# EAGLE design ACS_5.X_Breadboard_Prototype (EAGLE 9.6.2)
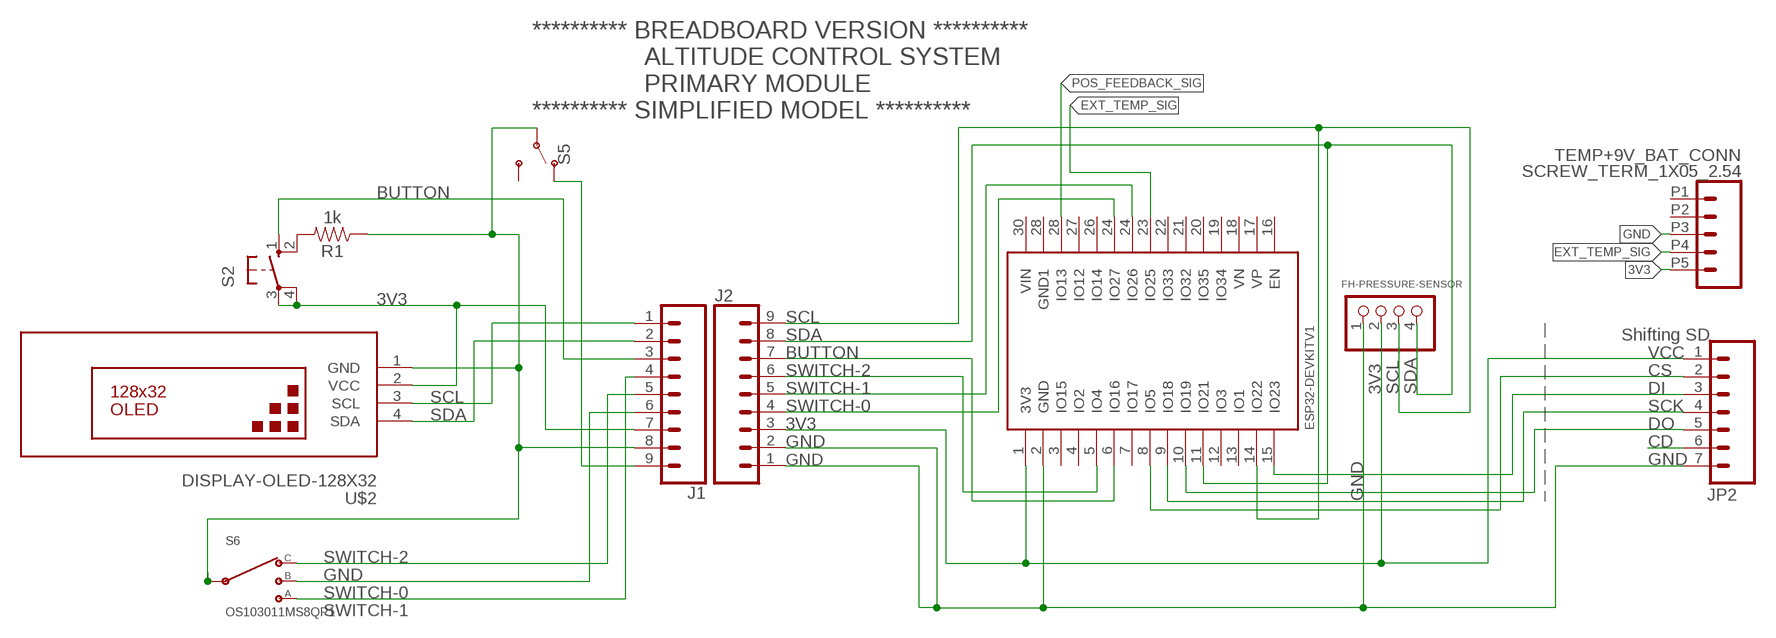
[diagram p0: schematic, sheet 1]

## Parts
FH-PRESSURE-SENSOR  PINHD-1X4  [1X04]
J1  CONN_09  [1X09]
J2  CONN_09  [1X09]
JP2  M07  [1X07]
R1  1k  1KOHM-HORIZ-1/4W-1%  [AXIAL-0.3]
S2  10-XX  [B3F-10XX]
S5  SWITCH-SPDT-PTH-11.6X4.0MM  [SWITCH_SPDT_PTH_11.6X4.0MM]
S6  OS103011MS8QP1  [OS102011MS8QP1]
TEMP+9V_BAT_CONN  SCREW_TERM_1X05_2.54  [1X05_2.54_SCREWTERM]
U$2  DISPLAY-OLED-128X32  [DISPLAY-OLED-128X32]
U$3  ESP32DEVKITV1  [ESP32-DEVKITV1]

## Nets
3V3: FH-PRESSURE-SENSOR.2 J1.7 J2.3 JP2.1 S2.3(P) S2.4(P1) TEMP+9V_BAT_CONN.P5 U$2.2(VCC) U$3.1(3V3)
BUTTON: J1.3 J2.7 S2.1(S) U$3.6(IO16)
EXT_TEMP_SIG: TEMP+9V_BAT_CONN.P4 U$3.23(IO25)
GND: FH-PRESSURE-SENSOR.1 J1.8 J2.1 J2.2 JP2.7 R1.P$1 S5.2(P) S6.2(C) TEMP+9V_BAT_CONN.P3 U$2.1(GND) U$3.2(GND)
N$1: R1.P$2 S2.2(S1)
N$4: J1.9 S5.1(O)
N$8: JP2.6
N$11: JP2.3 U$3.15(IO23)
N$12: JP2.2 U$3.8(IO5)
N$13: JP2.4 U$3.9(IO18)
N$14: JP2.5 U$3.10(IO19)
POS_FEEDBACK_SIG: U$3.28(IO13)
SCL: FH-PRESSURE-SENSOR.3 J1.1 J2.9 U$2.3(SCL) U$3.14(IO22)
SDA: FH-PRESSURE-SENSOR.4 J1.2 J2.8 U$2.4(SDA) U$3.11(IO21)
SWITCH-0: J1.6 J2.4 S6.3 U$3.24(IO27)
SWITCH-1: J1.5 J2.5 S6.4 U$3.24(IO26)
SWITCH-2: J1.4 J2.6 S6.1 U$3.5(IO4)
Unconnected: S5.3(S) TEMP+9V_BAT_CONN.P1 TEMP+9V_BAT_CONN.P2 U$3.3(IO15) U$3.4(IO2) U$3.7(IO17) U$3.12(IO3) U$3.13(IO1) U$3.16(EN) U$3.17(VP) U$3.18(VN) U$3.19(IO34) U$3.20(IO35) U$3.21(IO32) U$3.22(IO33) U$3.26(IO14) U$3.27(IO12) U$3.28(GND1) U$3.30(VIN)

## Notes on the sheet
- ********** BREADBOARD VERSION ********** 
                  ALTITUDE CONTROL SYSTEM
                  PRIMARY MODULE
  ********** SIMPLIFIED MODEL **********
- Shifting SD
- VCC
- CS
- DI
- SCK
- DO
- CD

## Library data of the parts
FH-PRESSURE-SENSOR = pinhead:PINHD-1X4: PIN HEADER
J1 J2 = SparkFun-Connectors:CONN_09: Multi connection point. Often used as Generic Header-pin footprint for 0.1 inch spaced/style header connections On any of the 0.1 inch spaced packages, you can populate with these: Break Away Headers - Straight (PRT-00116) Break Away Male Headers - Right Angle (PRT-00553) Female Headers (PRT-00115)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
JP2 = SparkFun-Connectors:M07: Header 7 Standard 7-pin 0.1" header. Use with straight break away headers (SKU : PRT-00116), right angle break away headers (PRT-00553), swiss pins (PRT-00743), machine pins (PRT-00117), and female headers (PRT-00115). NOTES ON THE VARIANTS LOCK and LOCK_LONGPADS... This footprint was designed to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
R1 = SparkFun-Resistors:1KOHM: 1kΩ resistor; PROD_ID: RES-12182
S2 = DC_LOAD_AU:10-XX: OMRON SWITCH; MPN: B3F-1000; OC_FARNELL: 176432; OC_NEWARK: 36M3542
S5 = SparkFun-Switches:SWITCH-SPDT: Single Pole, Double Throw (SPDT) Switch Single-pole, double-throw (SPDT) switch. Variant Overview SMD-AYZ0202 Surface Mount DPDT Switch (COM-00597) Used on e.g. LilyPad Arduino USB - ATmega32U4 Board PTH-11.6X4.0MM SPDT Mini Power Switch (COM-00102) Used on e.g. SparkFun Simon Says - Through-Hole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; PROD_ID: SWCH-08261; SF_SKU: COM-00102
S6 = OS103011MS8QP1:OS103011MS8QP1: Slide Switch SP3T Through Hole; AVAILABILITY: Unavailable; DESCRIPTION: Switch Slide ON ON ON SP3T Top Slide 0.1A 12VDC 10000Cycle PC Pins Bracket Mount/Through Hole Bulk; MF: C&K; MP: OS103011MS8QP1; PACKAGE: None; PRICE: None
TEMP+9V_BAT_CONN = Connectors-Terminal_Block:SCREW_TERM_1X05_2.54
U$2 = diy-modules:DISPLAY-OLED-128X32: 128x32 Dot Matrix OLED Module with I2C interface based on SSD1306 chip More details available here: http://www.tinyosshop.com/index.php?route=product/product&product_id=953 Schematic available here: http://www.tinyosshop.com/datasheet/OLED%2012832.pdf SSD1306 datasheet: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
U$3 = ESP32-DEVKITV1:ESP32DEVKITV1

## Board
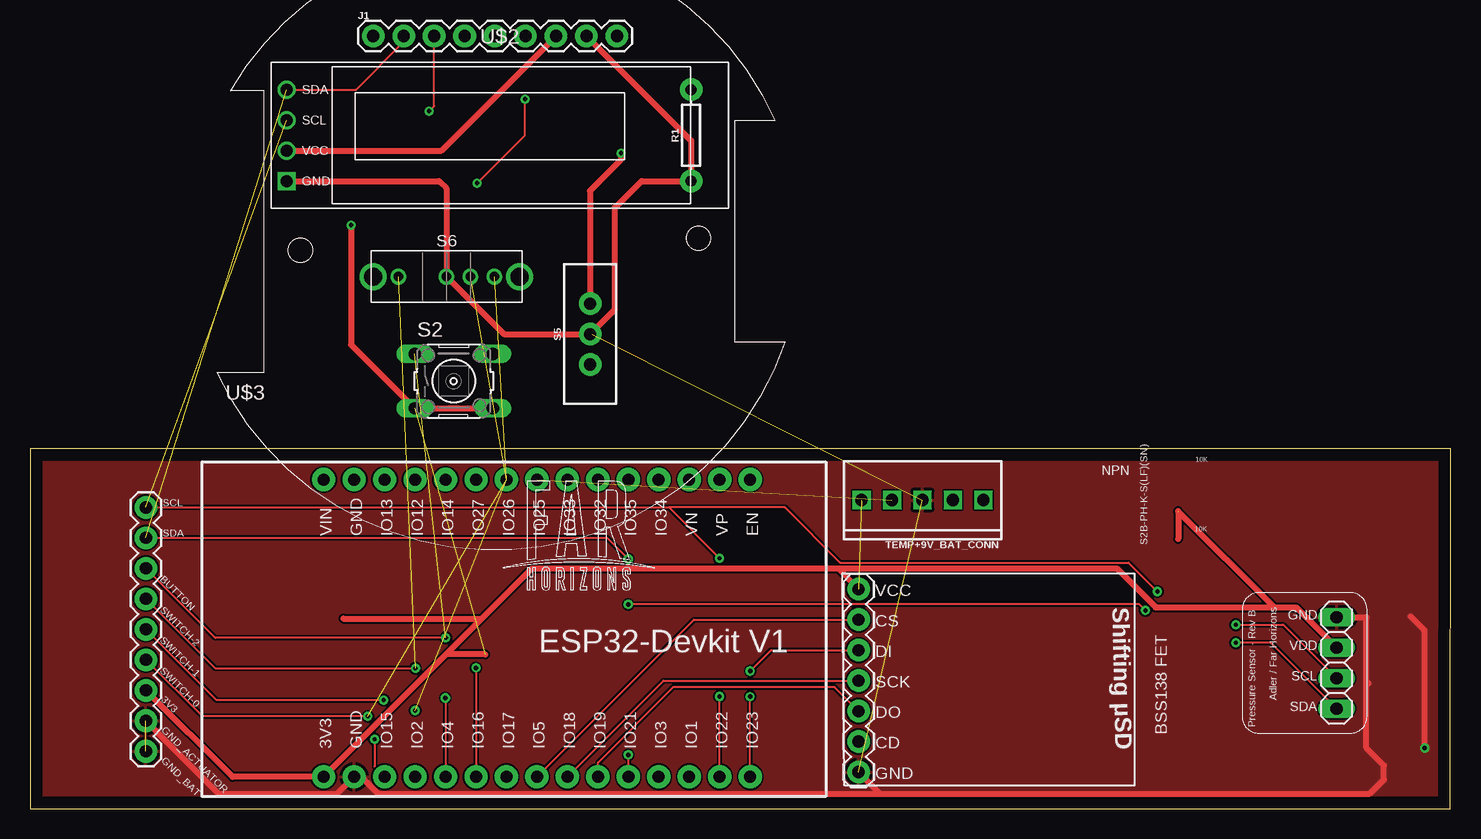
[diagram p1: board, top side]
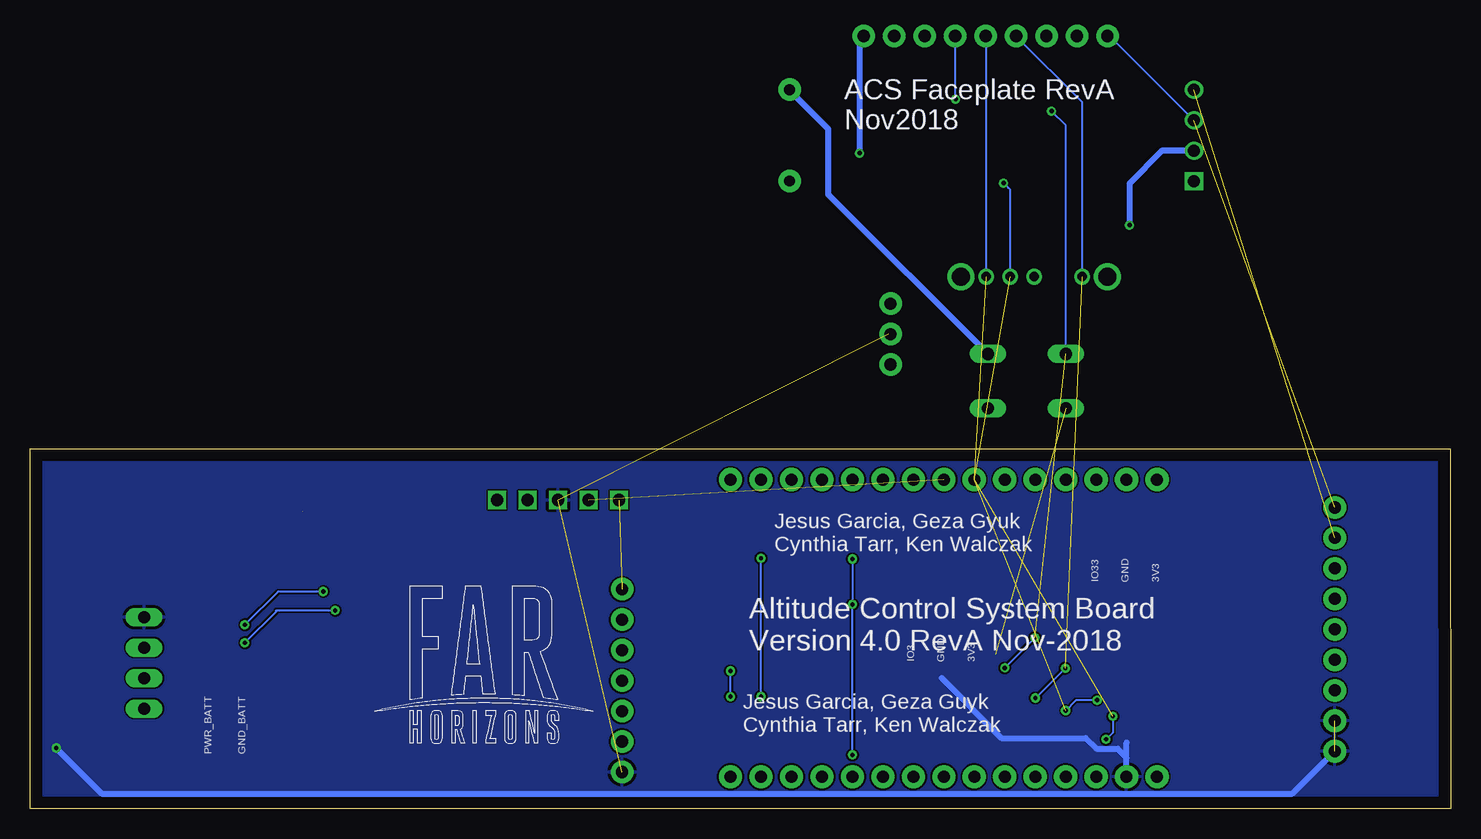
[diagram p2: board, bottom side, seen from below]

Size 118.43 x 30 mm. Coordinates in mm from the lower left corner, seen from the top.
Outline: 0,0 118.4,0 118.43,30 0.03,30 0,0
Copper layers (1*16): Top 0.035mm / dielectric 1.5mm / Bottom 0.035mm
Design rules "default": minimum track width 6mil, minimum drill 0.35mm, track to track 6mil, track to pad 6mil, pad to pad 6mil, via to via 6mil, smd to smd 6mil, copper to edge 40mil, drill to drill 6mil, minimum pad ring 10mil, minimum via ring 8mil, stop-mask expansion 4mil, vias tented up to drill 0mil, thermal gap 10mil

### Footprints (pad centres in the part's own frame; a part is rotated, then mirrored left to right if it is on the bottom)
1X04 = drill 1.016 long: 1 -3.81,0; 2 -1.27,0; 3 1.27,0; 4 3.81,0
1X09 = drill 1.016 pad 1.88: 1 0,0; 2 2.54,0; 3 5.08,0; 4 7.62,0; 5 10.16,0; 6 12.7,0; 7 15.24,0; 8 17.78,0; 9 20.32,0
1X07 = drill 1.016 pad 1.88: 1 0,0; 2 2.54,0; 3 5.08,0; 4 7.62,0; 5 10.16,0; 6 12.7,0; 7 15.24,0
AXIAL-0.3 = drill 0.9 pad 1.88: P$1 -3.81,0; P$2 3.81,0
B3F-10XX = drill 1.016 long: 1 -3.251,2.261; 2 3.251,2.261; 3 -3.251,-2.261; 4 3.251,-2.261
SWITCH_SPDT_PTH_11.6X4.0MM = drill 1.016 pad 1.88: 1 0,2.54; 2 0,0; 3 0,-2.54
OS102011MS8QP1 = drill 0.8: 1 -4,0; 2 0,0; 3 2,0; 4 4,0 | drill 1.5: MOUNT1 -6.1,0; MOUNT2 6.1,0
1X05_2.54_SCREWTERM = drill 1.016 square: P1 0,0; P2 2.54,0; P3 5.08,0; P4 7.62,0; P5 10.16,0
DISPLAY-OLED-128X32 = drill 1 square: 1 -17.78,-3.81 | drill 1: 2 -17.78,-1.27; 3 -17.78,1.27; 4 -17.78,3.81
ESP32-DEVKITV1 = drill 1 pad 1.93: 1 -22.87,-13.54; 2 -20.33,-13.54; 3 -17.79,-13.54; 4 -15.25,-13.54; 5 -12.71,-13.54; 6 -10.17,-13.54; 7 -7.63,-13.54; 8 -5.09,-13.54; 9 -2.55,-13.54; 10 -0.01,-13.54; 11 2.53,-13.54; 12 5.07,-13.54; 13 7.61,-13.54; 14 10.15,-13.54; 15 12.69,-13.54; 16 12.69,11.23; 17 10.15,11.23; 18 7.61,11.23; 19 5.07,11.23; 20 2.53,11.23; 21 -0.01,11.23; 22 -2.55,11.23; 23 -5.09,11.23; 24 -7.63,11.23; 25 -10.17,11.23; 26 -12.71,11.23; 27 -15.25,11.23; 28 -17.79,11.23; 29 -20.33,11.23; 30 -22.87,11.23

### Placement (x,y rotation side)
FH-PRESSURE-SENSOR  108.92,12.15 270 top
J1  28.61,64.39 0 top  (outside the outline)
J2  9.66,4.79 90 top
JP2  69.07,18.3 270 top
R1  55.11,56.12 90 top  (outside the outline)
S2  35.33,35.64 0 top  (outside the outline)
S5  46.7,39.56 0 top  (outside the outline)
S6  34.72,44.34 0 top  (outside the outline)
TEMP+9V_BAT_CONN  79.48,25.73 180 top
U$2  39.17,56.12 0 top  (outside the outline)
U$3  47.34,16.2 0 top

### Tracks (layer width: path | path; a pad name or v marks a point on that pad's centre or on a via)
3V3  (via drill 0.35)  (3 unrouted)
  Top 0.508: J2.3 16.88,2.65 U$3.1 34.67,12.86 | 34.67,12.86 37.66,15.85 | 37.66,15.85 41.84,20.03 67.34,20.03 | JP2.1 67.34,20.03 | 67.34,20.03 90.6,20.03 93.84,16.79 93.84,16.78 103.72,16.78 | 103.72,16.78 105.56,16.78 FH-PRESSURE-SENSOR.2 | 95.71,24.78 95.71,22.49 | 26.11,15.85 37.66,15.85 | 37.94,12.86 34.67,12.86 | 103.72,16.78 95.7,24.81 | U$2.2 34.31,54.85 J1.7 | v26.77,48.64 26.77,38.69 S2.3 S2.4
  Bottom 0.508: U$2.2 24.07,54.84 26.77,52.09 v26.77,48.64
BUTTON  (via drill 0.35)  (1 unrouted)
  Top 0.152: v37.17,11.74 U$3.6 | v34.66,14.25 15.44,14.25 J2.7 | v33.27,58.14 33.69,58.56 J1.3
  Bottom 0.152: v34.66,14.25 v37.17,11.74 | v33.27,58.14 32.08,56.95 S2.1
EXT_TEMP_SIG  (1 unrouted)
GND  (via drill 0.35)  (3 unrouted)
  Top 0.152: S5.2 46.82,39.56 46.85,39.56
  Top 0.508: J2.2 15.73,1.27 25.62,1.27 U$3.2 27.61,2.67 29.01,1.27 70.86,1.27 | 70.86,1.27 111.7,1.27 112.86,2.43 112.86,3.6 111.4,5.06 111.4,10.61 | JP2.7 70.86,1.27 | 111.56,10.45 111.4,10.61 | 111.4,10.61 111.4,15.95 111.39,15.96 FH-PRESSURE-SENSOR.1 | 115.07,16.04 116.25,14.86 v116.25,5.07 v116.25,5.06 | J1.8 55.11,55.67 R1.P$1 50.99,52.31 48.77,50.09 48.77,41.63 S5.2 | 46.82,39.56 39.5,39.56 S6.2 34.72,51.69 34.1,52.31 U$2.1
  Bottom 0.508: U$3.2 27.02,4.25 | 27.02,4.25 27.02,5.51 27,5.53 | 42.44,10.9 37.43,5.9 30.44,5.9 29.55,5.01 27.77,5.01 27.02,4.25 | v116.25,5.06 112.46,1.27 13.18,1.27 J2.1
  pour Top: -4.15,31.64 -4.15,-1.81 119.4,-1.81 119.4,31.64
  pour Bottom: -5.76,31.6 -5.76,-1.75 119.61,-1.75 119.61,31.6
N$1
  Bottom 0.508: S2.2 51.87,51.19 51.87,56.64 55.11,59.88 R1.P$2
N$4  (via drill 0.35)
  Top 0.508: v49.27,54.64 49.27,54.09 46.67,51.49 46.67,42.13 S5.1
  Bottom 0.508: J1.9 49.27,64.05 v49.27,54.64
N$11  (via drill 0.35)
  Top 0.152: U$3.15 v60.03,9.35 | v60.03,11.48 61.77,13.22 JP2.3
  Bottom 0.152: v60.03,9.35 v60.03,11.48
N$12
  Top 0.152: U$3.8 55.35,15.76 JP2.2
N$13
  Top 0.152: U$3.9 52.81,10.68 JP2.4
N$14
  Top 0.152: U$3.10 47.34,3.85 53.61,10.13 67.08,10.13 JP2.5
SCL  (via drill 0.35)  (1 unrouted)
  Top 0.152: U$3.14 v57.49,9.35 v57.49,9.36 | J2.9 53.25,25.11 | 53.25,25.11 v57.49,20.88 | v93.98,18.11 91.56,20.52 67.53,20.52 62.94,25.11 53.25,25.11 | v100.52,15.34 104.46,15.34 FH-PRESSURE-SENSOR.3
  Bottom 0.152: v93.98,18.11 97.75,18.11 v100.52,15.34 | v57.49,9.36 v57.49,20.88 | U$2.3 28.39,64.39 J1.1
SDA  (via drill 0.35)  (1 unrouted)
  Top 0.152: J2.8 48.12,22.57 | v92.98,16.53 92.48,17.03 v49.88,17.03 | FH-PRESSURE-SENSOR.4 103.43,13.83 v100.52,13.83 | v49.88,20.82 48.12,22.57 | 48.12,22.57 | U$3.11 v49.88,4.49 | U$2.4 27.17,59.93 31.15,63.91 J1.2
  Bottom 0.152: v100.52,13.83 97.91,16.44 97.91,16.53 v92.99,16.53 v92.98,16.53 | v49.88,20.82 v49.88,17.03 v49.88,4.49
SWITCH-0  (via drill 0.35)  (2 unrouted)
  Top 0.152: v28.16,7.7 14.38,7.7 J2.4 | v28.73,5.8 28.71,5.79 28.71,3.5 | v37.27,52.14 41.27,56.14 v41.27,59.14
  Bottom 0.152: v28.73,5.8 28.18,6.34 28.18,7.68 v28.16,7.7 | 36.87,51.74 v37.27,52.14 36.72,51.59 S6.3 | v41.27,59.14 41.27,64.35 J1.6
SWITCH-1  (via drill 0.35)  (2 unrouted)
  Top 0.152: v29.47,9.06 15.55,9.06 J2.5
  Bottom 0.152: v29.47,9.06 31.23,9.06 v32.09,8.19 | 38.87,64.29 J1.5 38.72,64.34 S6.4
SWITCH-2  (via drill 0.35)  (1 unrouted)
  Top 0.152: v34.62,9.23 34.62,2.67 U$3.5 | J2.6 15.43,11.72 v32.13,11.72
  Bottom 0.152: v34.62,9.23 v32.13,11.72 | J1.4 30.72,58.88 S6.1

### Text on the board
tPlace: Shifting µSD
bPlace: ACS Faceplate RevA / Nov2018 | Jesus Garcia, Geza Gyuk / Cynthia Tarr, Ken Walczak | Altitude Control System Board / Version 4.0 RevA Nov-2018 | Jesus Garcia, Geza Guyk / Cynthia Tarr, Ken Walczak
tNames: 10K | NPN | SCL | SDA | 10K | S2B-PH-K-S(LF)(SN) | BUTTON | VCC | SWITCH-2 | Pressure Sensor - Rev B | Adler / Far Horizons | GND | CS | SWITCH-1 | VDD | DI | SWITCH-0 | SCL | SCK | 3V3 | SDA | DO | GND_ACTUATOR | BSS138 FET | CD | GND_BAT | GND
bNames: GND | IO33 | 3V3 | 3V3 | GND | IO3 | GND_BATT | PWR_BATT
tValues: 10uF | 0.33uF
Measures: center: 19.59
Document: Measurements of: / - OLED 38.11 x 12 mm / - Switch (3) 17 x 6 mm OS103011MS8QP1 / - Switch (2) 3.8 x 8.6 mm / - Button 6.15 x 6.15 mm / - Size of Screw Hole / - 3mm floors / / Location of Hole(s) made with Vias / Dimension Constraints 50mm diameter / Location of Part Placement / Abs Center to 9pin connector: 17.25

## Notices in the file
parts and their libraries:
SparkFun-Connectors: Licensing: Creative Commons ShareAlike 4.0 International - https://creativecommons.org/licenses/by-sa/4.0
SparkFun-Connectors: Licensing: CC v3.0 Share-Alike You are welcome to use this library for commercial purposes.
